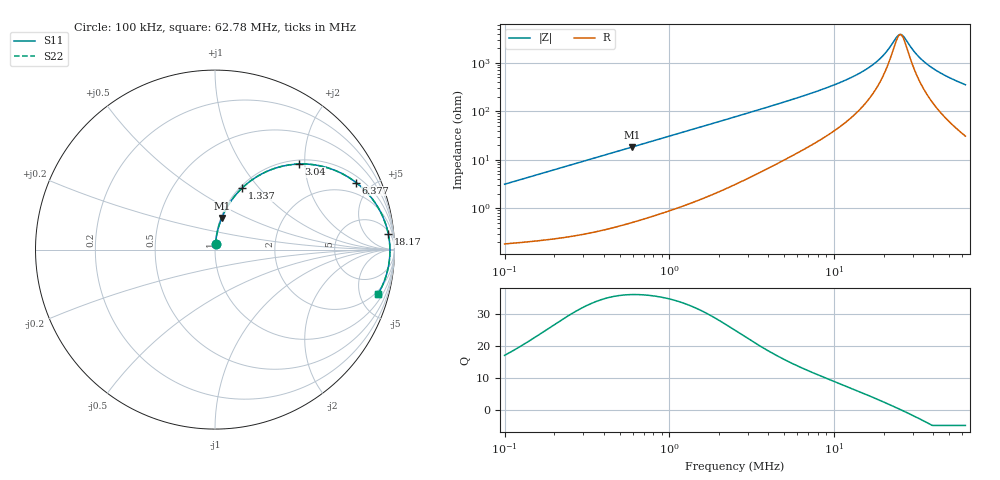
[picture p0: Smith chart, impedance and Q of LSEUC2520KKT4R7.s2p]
! LSEUC2520KKT4R7  S-PARAMETER MODEL  ( General Type )
! Model Generated by TAIYO YUDEN Corporation (http://www.ty-top.com)
! Version 1.0
! TAIYO YUDEN Control No. 211126
! Copyright(c) 2021 TAIYO YUDEN CO.,LTD. All Rights Reserved.
! Product Description (link to TY-COMPAS)
! https://ds.yuden.co.jp/TYCOMPAS/or/detail?pn=LSEUC2520KKT4R7M&u=M
! Products Name : Inductors
! Characteristics :
!  Inductance : 4.7 uH , SRF(min) : -Hz , DC Resistance(max) : 0.16 Ohm
!  Rated Current : Saturation :2200 mA , Temp Rise : 1800 mA (40 degC)
!  Case Size : 2.5 x 2.0 / 0.098 x 0.079 [mm/inch] , Thickness : 1 / 0.039 [mm/inch]
!  (Conditions: Temperature = 25 degC , DC Bias Current/Voltage = 0A / 0V)
! External Node Assignments :
!  1  o---GGG---o  2
! GND o---------o GND
! Frequency Range : 0.1MHz  -  62.782943MHz  [ 402 STEP ]
# MHz S RI R 50
! Freq[MHz].  S11 Real  S11 Imag  S21 Real  S21 Imag  S12 Real  S12 Imag  S22 Real  S22 Imag
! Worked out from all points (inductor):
!   401 points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, 100 kHz to 62.78 MHz, reference 50 ohm
!   read as one part in series: L = 4.96 uH near 103.3 kHz
!   highest Q = 36.1 at 597.6 kHz (marker M1), where L = 4.9 uH
!   self-resonance near 25.28 MHz
!   S11 on the Smith chart (normalised r, x): 100 kHz: 1.00, +0.06; 1.337 MHz: 1.03, +0.82; 3.04 MHz: 1.08, +1.86; 6.377 MHz: 1.31, +4.05; 18.17 MHz: 7, +20; 62.78 MHz: 1.61, -7.03
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0.1  0.0028 0.0311  0.9972 -0.0311  0.9972 -0.0311  0.0028 0.0311
0.294197  0.011 0.0898  0.989 -0.0898  0.989 -0.0898  0.011 0.0898
0.597587  0.0373 0.1761  0.9627 -0.1761  0.9627 -0.1761  0.0373 0.1761
0.86552  0.0718 0.2444  0.9282 -0.2444  0.9282 -0.2444  0.0718 0.2444
1.337  0.1507 0.3427  0.8493 -0.3427  0.8493 -0.3427  0.1507 0.3427
1.815636  0.2428 0.412  0.7572 -0.412  0.7572 -0.412  0.2428 0.412
2.546334  0.3824 0.4661  0.6176 -0.4661  0.6176 -0.4661  0.3824 0.4661
3.039878  0.4665 0.4768  0.5335 -0.4768  0.5335 -0.4768  0.4665 0.4768
4.263269  0.6281 0.4557  0.3719 -0.4557  0.3719 -0.4557  0.6281 0.4557
6.376875  0.7872 0.3728  0.2128 -0.3728  0.2128 -0.3728  0.7872 0.3728
7.371558  0.831 0.3343  0.169 -0.3343  0.169 -0.3343  0.831 0.3343
12.74606  0.9362 0.1804  0.0638 -0.1804  0.0638 -0.1804  0.9362 0.1804
15.46362  0.9553 0.1279  0.0447 -0.1279  0.0447 -0.1279  0.9553 0.1279
18.16591  0.9658 0.0853  0.0342 -0.0853  0.0342 -0.0853  0.9658 0.0853
21.68692  0.9725 0.0393  0.0275 -0.0393  0.0275 -0.0393  0.9725 0.0393
24.27504  0.9744 0.0104  0.0256 -0.0104  0.0256 -0.0104  0.9744 0.0104
25.0697  0.9746 0.00211  0.0254 -0.00211  0.0254 -0.00211  0.9746 0.00211
25.89038  0.9747 -0.00617  0.0253 0.00617  0.0253 0.00617  0.9747 -0.00617
31.41042  0.972 -0.0562  0.028 0.0562  0.028 0.0562  0.972 -0.0562
36.89944  0.9654 -0.0988  0.0346 0.0988  0.0346 0.0988  0.9654 -0.0988
46.98279  0.9469 -0.1654  0.0531 0.1654  0.0531 0.1654  0.9469 -0.1654
62.78294  0.9071 -0.2498  0.0929 0.2498  0.0929 0.2498  0.9071 -0.2498
